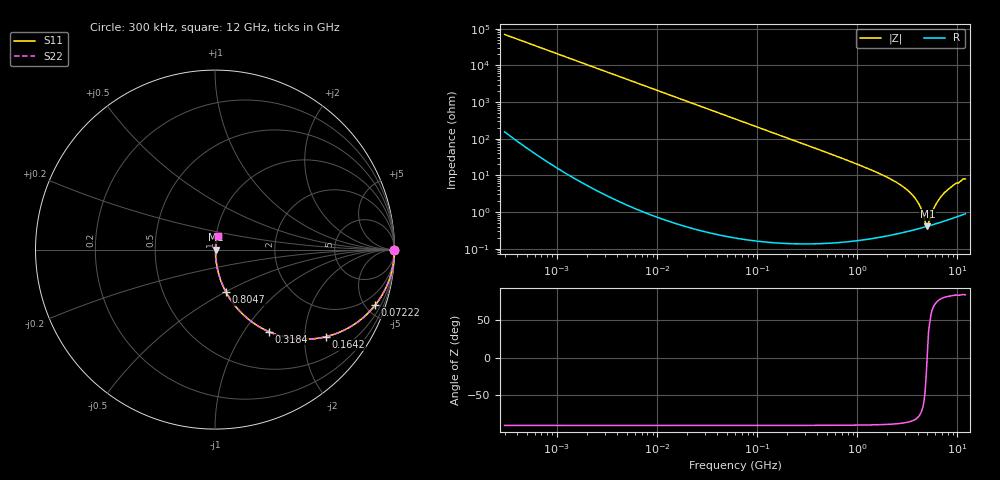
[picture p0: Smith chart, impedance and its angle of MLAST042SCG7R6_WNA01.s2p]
! MLAST042SCG7R6_WNA01  S-PARAMETER MODEL  ( General Type )
! Model Generated by TAIYO YUDEN Corporation (http://www.ty-top.com)
! Version 1.0
! TAIYO YUDEN Control No. 150820
! Copyright(c) 2015 TAIYO YUDEN CO.,LTD. All Rights Reserved.
! Product Description (link to TY-COMPAS)
! https://ds.yuden.co.jp/TYCOMPAS/or/detail?pn=MLAST042SCG7R6BWNA01&u=M
! Products Name : Multilayer Ceramic Capacitors
! Characteristics :
!  Capacitance : 7.6 pF , Rated Voltage : 25V , TCC : CG / C0G
!  Case Size : 0.4 x 0.2 / 0.016 x 0.008 [mm/inch] , Thickness : 0.2 / 0.008 [mm/inch]
!  (Conditions: Temperature = 25 degC , DC Bias Current/Voltage = 0A / 0V)
! External Node Assignments :
!  1  o---| |---o  2
! GND o---------o GND
! Frequency Range : 0.3MHz  -  12000MHz  [ 401 STEP ]
# MHz S RI R 50
! Freq[MHz].  S11 Real  S11 Imag  S21 Real  S21 Imag  S12 Real  S12 Imag  S22 Real  S22 Imag
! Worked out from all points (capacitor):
!   401 points, 300 kHz to 12 GHz, reference 50 ohm
!   read as one part in series: C = 7.62 pF near 316.3 kHz
!   lowest |Z| = 409 mohm at 5.006 GHz (marker M1)
!   series resonance near 4.978 GHz, so ESL is about 130 pH
!   S11 on the Smith chart (normalised r, x): 300 kHz: open; 72.22 MHz: 1.00, -5.78; 164.2 MHz: 1.00, -2.54; 318.4 MHz: 1.00, -1.31; 804.7 MHz: 1.00, -0.51; 12 GHz: 1.02, +0.16
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0.3  1 -0.00144  5.22e-06 0.00144  5.22e-06 0.00144  1 -0.00144
1.769972  0.9999 -0.00847  7.63e-05 0.00847  7.63e-05 0.00847  0.9999 -0.00847
10.44266  0.9975 -0.0499  0.00251 0.0499  0.00251 0.0499  0.9975 -0.0499
27.10171  0.9834 -0.1276  0.0166 0.1276  0.0166 0.1276  0.9834 -0.1276
60  0.9236 -0.2653  0.0764 0.2653  0.0764 0.2653  0.9236 -0.2653
72.22496  0.893 -0.3088  0.107 0.3088  0.107 0.3088  0.893 -0.3088
107.4644  0.7904 -0.4066  0.2096 0.4066  0.2096 0.4066  0.7904 -0.4066
164.1901  0.6175 -0.4854  0.3825 0.4854  0.3825 0.4854  0.6175 -0.4854
318.4019  0.2996 -0.457  0.7004 0.457  0.7004 0.457  0.2996 -0.457
353.9943  0.2568 -0.4357  0.7432 0.4357  0.7432 0.4357  0.2568 -0.4357
804.7407  0.0613 -0.2369  0.9387 0.2369  0.9387 0.2369  0.0613 -0.2369
2088.533  0.00897 -0.0815  0.991 0.0815  0.991 0.0815  0.00897 -0.0815
2870.14  0.00507 -0.0482  0.9949 0.0482  0.9949 0.0482  0.00507 -0.0482
3642.919  0.00391 -0.0264  0.9961 0.0264  0.9961 0.0264  0.00391 -0.0264
4158.869  0.00375 -0.0151  0.9963 0.0151  0.9963 0.0151  0.00375 -0.0151
4747.894  0.0039 -0.00394  0.9961 0.00394  0.9961 0.00394  0.0039 -0.00394
5006.236  0.00405 0.000468  0.996 -0.000468  0.996 -0.000468  0.00405 0.000468
5140.631  0.00414 0.00278  0.9959 -0.00278  0.9959 -0.00278  0.00414 0.00278
6026.253  0.0049 0.0143  0.9951 -0.0143  0.9951 -0.0143  0.0049 0.0143
7064.448  0.00616 0.028  0.9938 -0.028  0.9938 -0.028  0.00616 0.028
9207.246  0.00974 0.0536  0.9903 -0.0536  0.9903 -0.0536  0.00974 0.0536
12000  0.015 0.0775  0.985 -0.0775  0.985 -0.0775  0.015 0.0775
